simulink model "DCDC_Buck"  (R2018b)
settings: Solver=FixedStepDiscrete  StartTime=0.0  StopTime=Inf  RelTol=1e-3  EnableMultiTasking=on
undefined symbols (not defined in the file): A, ADCIN0, ADCIN1, ADCINA0, ADCINB0, bit, Compare, conversion, DCAEVT1, DCAEVT1FILT, Digital, ended, Event, Filtered, GPTRIP1SEL, GPTRIP2SEL, hex2dec, input, Module, of, Single, start, Trip, TZ1, TZ2, version, Zone
libraries: c2837xDlib x3, c2802xlib x3, tiiqmathlib x2, c280xlib x2, c2000lib x1, demo_controls x1, simulink x1

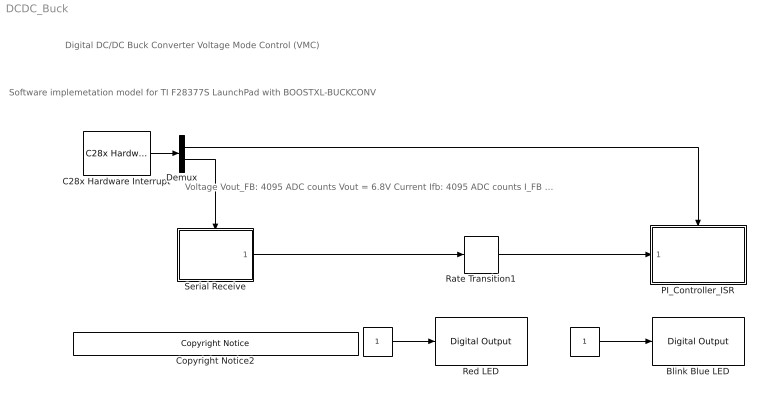
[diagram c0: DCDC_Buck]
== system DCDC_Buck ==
  note: Voltage Vout_FB: 4095 ADC counts Vout = 6.8V Current Ifb: 4095 ADC counts I_FB = 3.3A
  note: Software implemetation model for TI F28377S LaunchPad with BOOSTXL-BUCKCONV
  note: Digital DC/DC Buck Converter Voltage Mode Control (VMC)
  " " : Constant  OutDataTypeStr=uint16  SampleTime=0.5
  "   " : Constant  OutDataTypeStr=uint16  SampleTime=0.5
  Blink Blue LED : c2837xDlib/Digital Output  GPIO_Number=GPIO8~GPIO15  GPIO_Bit0=off  GPIO_BIT0_Toggle=off  GPIO_Bit1=off  GPIO_BIT1_Toggle=off  GPIO_Bit2=off  GPIO_BIT2_Toggle=off  GPIO_Bit3=off  GPIO_BIT3_Toggle=off  GPIO_Bit4=off  GPIO_BIT4_Toggle=on  GPIO_Bit5=on  GPIO_BIT5_Toggle=on  GPIO_Bit6=off  GPIO_BIT6_Toggle=off  GPIO_Bit7=off  GPIO_BIT7_Toggle=off
  C28x Hardware Interrupt : c2000lib/Scheduling/C28x Hardware Interrupt  irqnumbers=[1 9]  pienumbers=[1 1]  irqpriorities=[30 50]  irqpreempts=[0 1]  showinput=off  dspchiptype=C280X
  Copyright Notice2 : demo_controls/Copyright Notice  year=2017  prod=tic2000
  Demux : Demux  Outputs=2
  PI_Controller_ISR : Subsystem
  Rate Transition1 : RateTransition  Integrity=off
  Red LED : c2837xDlib/Digital Output  GPIO_Number=GPIO8~GPIO15  GPIO_Bit0=off  GPIO_BIT0_Toggle=off  GPIO_Bit1=off  GPIO_BIT1_Toggle=off  GPIO_Bit2=off  GPIO_BIT2_Toggle=off  GPIO_Bit3=off  GPIO_BIT3_Toggle=off  GPIO_Bit4=on  GPIO_BIT4_Toggle=off  GPIO_Bit5=off  GPIO_BIT5_Toggle=on  GPIO_Bit6=off  GPIO_BIT6_Toggle=off  GPIO_Bit7=off  GPIO_BIT7_Toggle=off
  Serial Receive : Subsystem  SystemSampleTime=1e-3
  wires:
  Serial Receive/1(Out1) -> Rate Transition1/1
  " "/1 -> Blink Blue LED/1
  Demux/1 -> PI_Controller_ISR/Trigger
  Demux/2 -> Serial Receive/Trigger
  C28x Hardware Interrupt/1 -> Demux/1
  Rate Transition1/1 -> PI_Controller_ISR/1(Voltage/P/I Demand)
  "   "/1 -> Red LED/1

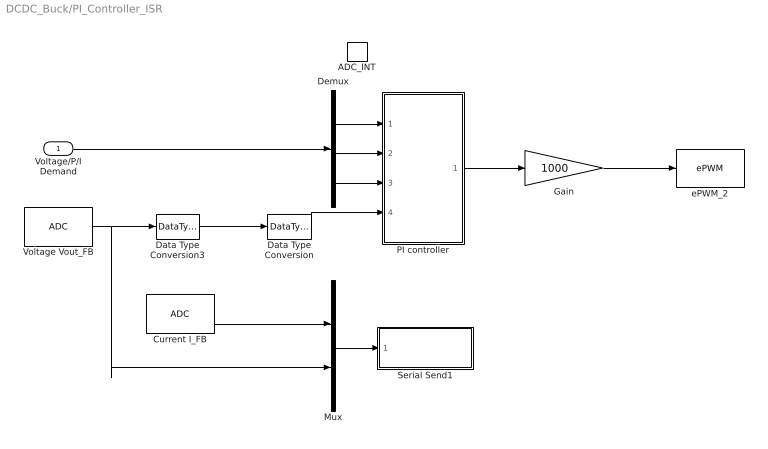
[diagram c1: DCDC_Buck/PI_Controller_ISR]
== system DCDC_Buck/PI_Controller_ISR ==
  Voltage/P/I Demand : Inport
  ADC_INT : TriggerPort  TriggerType=function-call  VariantControl=Variant  PortDimensions=1
  Current I_FB : c2802xlib/ADC  ADCModule=A  samplingMode=Single sample mode  ADCResolution=12-bit (Single-ended input)  useSOC1=SOC1  useSOC2=SOC0_SOC1  SOCAcquisitionWindow=14  SOCTriggerSource=ePWM2_ADCSOCA  SOCInterruptTrigger=No ADCINT  Ts=-1  dType=uint16  postInterrupt=off  interruptSel=ADCINT1  ADCINTContinuous=on  endma=off  chdma=1  blkParamProc=C2000_Type4  conv1=ADCINA0  conv2=ADCINA0 and ADCINB0  conv1_Type4=ADCIN2  conv2_Type4=ADCIN0 and ADCIN1
  Data Type Conversion : DataTypeConversion  OutDataTypeStr=fixdt(1,32,24)  RndMeth=Simplest
  Data Type Conversion3 : DataTypeConversion  OutDataTypeStr=fixdt(0,16,12)  ConvertRealWorld=Stored Integer (SI)  RndMeth=Simplest
  Demux : Demux  Outputs=3
  Gain : Gain  Gain=1000  ParamDataTypeStr=int16  OutDataTypeStr=fixdt(1,32,20)  RndMeth=Simplest
  Mux : Mux  Inputs=2
  PI controller : Subsystem
  Serial Send1 : Subsystem
  Voltage Vout_FB : c2802xlib/ADC  ADCModule=A  samplingMode=Single sample mode  ADCResolution=12-bit (Single-ended input)  useSOC1=SOC0  useSOC2=SOC0_SOC1  SOCAcquisitionWindow=14  SOCTriggerSource=ePWM2_ADCSOCA  SOCInterruptTrigger=No ADCINT  Ts=-1  dType=uint16  postInterrupt=on  interruptSel=ADCINT1  ADCINTContinuous=on  endma=off  chdma=1  blkParamProc=C2000_Type4  conv1=ADCINA0  conv2=ADCINA0 and ADCINB0  conv1_Type4=ADCIN3  conv2_Type4=ADCIN0 and ADCIN1
  ePWM_2 : c2802xlib/ePWM  useModule=ePWM2  ePWMxLINKTBPRD=Not Linked  periodUnits=Clock cycles  timerSource=Specify via dialog  timerPeriod_clk=1000  timerPeriod_sec=0.0001  tbshadow=Counter equals to zero  countingMode=Up  phaseActiveEnable=Disable  phaseDirection=Count down after sync  phaseActive=0  synchronizationEnable=off  dcaevt1Sync=off  dcbevt1Sync=off  synchronizationOption=Disable  clockPrescale=1  HSclockPrescale=1  enswap=off  ePWMxAStatus=on  ePWMxAactionLogic1=Set  ePWMxAactionLogic2=Do nothing  ePWMxAactionLogic3=Clear  ePWMxAactionLogic4=Set  ePWMxAactionLogic5=Do nothing  ePWMxAactionLogic6=Do nothing  ePWMxALoadMode=Load on counter equals to period (CTR=PRD)  ePWMxACSFenable=off  ePWMxACSFvalue=Forcing disable  ePWMxASFreload=Zero  ePWMxBStatus=off  ePWMxBactionLogic1=Set  ePWMxBactionLogic2=Clear  ePWMxBactionLogic3=Do nothing  ePWMxBactionLogic4=Do nothing  ePWMxBactionLogic5=Clear  ePWMxBactionLogic6=Set  ePWMxBLoadMode=Load on counter equals to zero (CTR=Zero)  ePWMxBCSFenable=off  ePWMxBCSFvalue=Forcing disable  ePWMxBSFreload=Zero  ePWNxBOutWay=off  ePWMxLINKCMPA=Not Linked  CMPAUnits=Clock cycles  CMPASource=Input port  CMPAValue_per=50  CMPAValue_clk=0  enCMPAshadow=Counter equals to zero  ePWMxLINKCMPB=Not Linked  CMPBUnits=Clock cycles  CMPBSource=Specify via dialog  CMPBValue_per=50  CMPBValue_clk=1000-((15+54)*2)  enCMPBshadow=Counter equals to zero  ePWMxLINKCMPC=Not Linked  CMPCUnits=Clock cycles  CMPCSource=Specify via dialog  CMPCValue_per=50  CMPCValue_clk=32000  enCMPCshadow=Counter equals to zero  ePWMxLINKCMPD=Not Linked  CMPDUnits=Clock cycles  CMPDSource=Specify via dialog  CMPDValue_per=50  CMPDValue_clk=32000  enCMPDshadow=Counter equals to zero  enableDBePWMxA=on  enableDBePWMxB=on  enhalfcycle=off  DBpolarity=Active high complementary (AHC)  DBedgeDelay=Positive  DBSource_ePWMxA=ePWMxA  DBSource_ePWMxB=ePWMxA  DBperiodSource=Specify via dialog  REDperiod=20  FEDperiod=20  adcstartModuleA=on  adcrequestEventA=First event  adcstartEventA=Digital Compare Module A Event 1 start of conversion (DCAEVT1.soc)  adcstartEventA_type2=Counter is incrementing and equals to the compare B register (CTRU=CMPB)  adcstartModuleB=off  adcrequestEventB=First event  adcstartEventB=Counter equals to zero (CTR=Zero)  adcstartEventB_type2=Counter equals to zero (CTR=Zero)  intEn=off  intPrd=First event  intSel=Counter equals to zero (CTR=Zero)  intSel_type2=Counter equals to zero (CTR=Zero)  hrpe=off  enHRPWM=off  HRPWM_LoadMode=Counter equals to period (CTR=PRD)  HRPWM_CTLMode=Duty or Period control mode  HRPWM_EDGMode=Both edge  hrpeb=off  enHRPWMB=off  HRPWM_LoadModeB=Counter equals to zero (CTR=ZERO)  HRPWM_CTLModeB=Duty or Period control mode  HRPWM_EDGModeB=Both edge  enSFO=on  enautoconv=on  chopperEnable=off  chopperFrequency=1  chopperFirstwidth=1  chopperDuty=12.5%  tripZonesource=Specify via dialog  tzselOSHT1=off  tzselOSHT2=off  tzselOSHT3=off  tzselOSHDCAEV1=off  tzselOSHDCBEV1=off  tzselCBC1=off  tzselCBC2=off  tzselCBC3=off  tzselCBCDCAEV2=off  tzselCBCDCBEV2=off  tzselOSHT4=off  tzselOSHT5=off  tzselOSHT6=off  tzselCBC4=off  tzselCBC5=off  tzselCBC6=off  enTzOstIntr=off  enTzCbcIntr=off  enTzDCAEVT1Intr=off  enTzDCAEVT2Intr=off  enTzDCBEVT1Intr=off  enTzDCBEVT2Intr=off  ePWMxAforced=No action  ePWMxBforced=No action  DCAEVT1forced=No action  DCBEVT1forced=No action  DCAEVT2forced=No action  DCBEVT2forced=No action  dcah=Trip Zone 1 input (TZ1)  dcal=Trip Zone 2 input (TZ2)  dcbh=Trip Zone 1 input (TZ1)  dcbl=Trip Zone 2 input (TZ2)  dcah_type2=GPTRIP1SEL/(TZ1)  dcal_type2=GPTRIP2SEL/(TZ2)  dcbh_type2=GPTRIP1SEL/(TZ1)  dcbl_type2=GPTRIP2SEL/(TZ2)  gendcaevt1=Event disabled  gendcaevt2=Event disabled  gendcbevt1=Event disabled  gendcbevt2=Event disabled  dcaevt1src=DCAEVT1 with sync  dcaevt2src=DCAEVT2 with sync  dcbevt1src=DCBEVT1 with sync  dcbevt2src=DCBEVT2 with sync  pulsesel=Counter equals to zero (CTR=Zero)  blankinv=off  blankoffset=0  blankwidth=0  evsrcsel=Filtered version of DCAEVT1 (DCAEVT1FILT)  encape=off  PwmType=C2000_Type4
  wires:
  Data Type Conversion3/1 -> Data Type Conversion/1
  Gain/1 -> ePWM_2/1
  PI controller/1(Duty1) -> Gain/1
  Data Type Conversion/1 -> PI controller/4(Vout1)
  Mux/1 -> Serial Send1/1(In1)
  Demux/1 -> PI controller/1(Vout1Ref)
  Demux/2 -> PI controller/2(P gain)
  Demux/3 -> PI controller/3(I gain)
  Voltage/P/I Demand/1 -> Demux/1
  Current I_FB/1 -> Mux/1
  Voltage Vout_FB/1 -> Mux/2, Data Type Conversion3/1

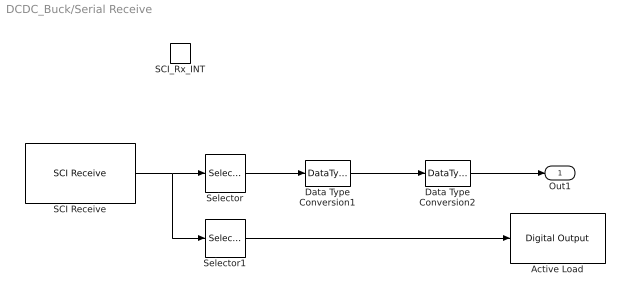
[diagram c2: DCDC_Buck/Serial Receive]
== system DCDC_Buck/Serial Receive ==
  SCI_Rx_INT : TriggerPort  TriggerType=function-call  VariantControl=Variant
  Active Load : c2837xDlib/Digital Output  GPIO_Number=GPIO16~GPIO23  GPIO_Bit0=off  GPIO_BIT0_Toggle=off  GPIO_Bit1=off  GPIO_BIT1_Toggle=off  GPIO_Bit2=on  GPIO_BIT2_Toggle=off  GPIO_Bit3=off  GPIO_BIT3_Toggle=off  GPIO_Bit4=off  GPIO_BIT4_Toggle=on  GPIO_Bit5=off  GPIO_BIT5_Toggle=off  GPIO_Bit6=off  GPIO_BIT6_Toggle=off  GPIO_Bit7=off  GPIO_BIT7_Toggle=off
  Data Type Conversion1 : DataTypeConversion  OutDataTypeStr=fixdt(0,16,14)  ConvertRealWorld=Stored Integer (SI)  RndMeth=Simplest
  Data Type Conversion2 : DataTypeConversion  OutDataTypeStr=fixdt(1,32,24)  RndMeth=Simplest
  SCI Receive : c280xlib/SCI Receive  sciModule=A  dataHead='S'  dataTail='E'  dataType=uint16  dataDim=4  initValue=0  errOption=Output the last received value  errValue=0  sampleTime=-1  outputStatus=off  postInterrupt=on  numFifo=10
  Selector : Selector  InputPortWidth=4  IndexOptions=Index vector (dialog)  Indices=[1 2 3]  OutputSizes=1
  Selector1 : Selector  InputPortWidth=4  IndexOptions=Index vector (dialog)  Indices=4  OutputSizes=1
  Out1 : Outport  InitialOutput=[0 0.002 0.003]
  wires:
  SCI Receive/1 -> Selector1/1, Selector/1
  Selector/1 -> Data Type Conversion1/1
  Selector1/1 -> Active Load/1
  Data Type Conversion1/1 -> Data Type Conversion2/1
  Data Type Conversion2/1 -> Out1/1

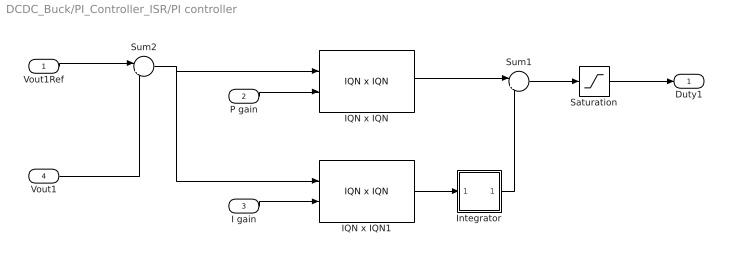
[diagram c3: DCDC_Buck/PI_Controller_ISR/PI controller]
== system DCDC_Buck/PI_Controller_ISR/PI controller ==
  Vout1Ref : Inport
  P gain : Inport  Port=2
  I gain : Inport  Port=3
  Vout1 : Inport  Port=4
  IQN x IQN : tiiqmathlib/IQN x IQN  multiplyOption=Multiply
  IQN x IQN1 : tiiqmathlib/IQN x IQN  multiplyOption=Multiply
  Integrator : Subsystem
  Saturation : Saturate  UpperLimit=0.6  LowerLimit=0  RndMeth=Simplest
  Sum1 : Sum  Inputs=|++  RndMeth=Simplest
  Sum2 : Sum  Inputs=|+-  RndMeth=Simplest
  Duty1 : Outport
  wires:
  P gain/1 -> IQN x IQN/2
  Vout1Ref/1 -> Sum2/1
  Integrator/1(y) -> Sum1/2
  Vout1/1 -> Sum2/2
  Sum2/1 -> IQN x IQN/1, IQN x IQN1/1
  I gain/1 -> IQN x IQN1/2
  Sum1/1 -> Saturation/1
  Saturation/1 -> Duty1/1
  IQN x IQN/1 -> Sum1/1
  IQN x IQN1/1 -> Integrator/1(u)

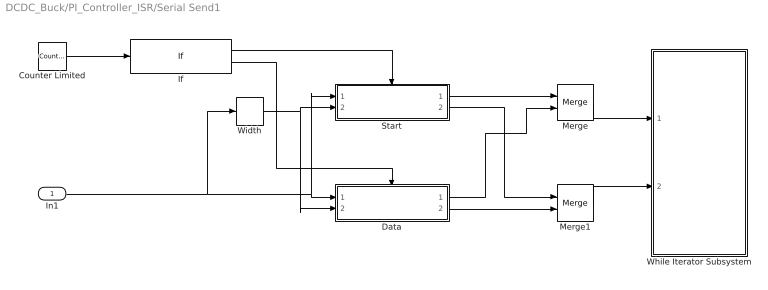
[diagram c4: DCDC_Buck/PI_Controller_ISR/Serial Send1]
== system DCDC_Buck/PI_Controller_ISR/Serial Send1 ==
  In1 : Inport
  Counter Limited : simulink/Sources/Counter Limited  uplimit=11999  tsamp=-1
  Data : Subsystem  TreatAsAtomicUnit=on
  If : If  IfExpression=u1 == 0
  Merge : Merge
  Merge1 : Merge
  Start : Subsystem  TreatAsAtomicUnit=on
  While Iterator Subsystem : Subsystem  TreatAsAtomicUnit=on
  Width : Width  OutDataTypeMode=All ports same datatype  DataType=uint16
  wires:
  If/1 -> Start/Action
  If/2 -> Data/Action
  Counter Limited/1 -> If/1
  Start/1(Data_out) -> Merge/1
  Data/1(Data_out) -> Merge/2
  Merge/1 -> While Iterator Subsystem/1(Data)
  Merge1/1 -> While Iterator Subsystem/2(Iteration)
  Start/2(Iteration) -> Merge1/1
  Data/2(Iteration) -> Merge1/2
  Width/1 -> Data/2(Data_width), Start/2(Data_width)
  In1/1 -> Width/1, Start/1(Data), Data/1(Data)

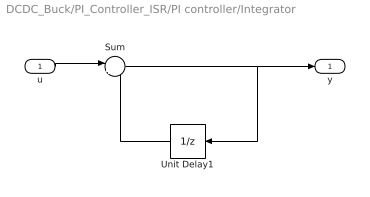
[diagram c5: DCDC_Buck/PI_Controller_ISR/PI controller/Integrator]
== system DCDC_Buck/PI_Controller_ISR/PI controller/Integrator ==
  u : Inport
  Sum : Sum  Inputs=|++  RndMeth=Simplest
  Unit Delay1 : UnitDelay  SampleTime=-1
  y : Outport
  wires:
  Sum/1 -> Unit Delay1/1, y/1
  Unit Delay1/1 -> Sum/2
  u/1 -> Sum/1

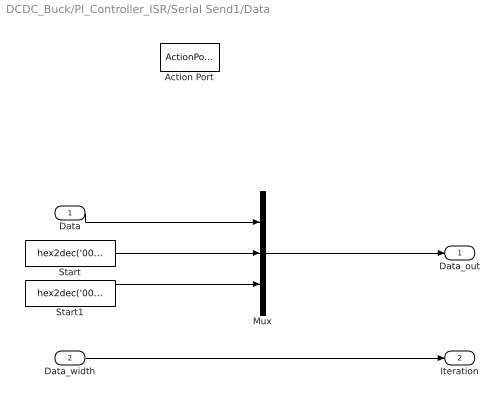
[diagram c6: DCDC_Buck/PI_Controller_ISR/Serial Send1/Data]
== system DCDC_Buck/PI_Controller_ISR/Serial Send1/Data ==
  Data : Inport
  Data_width : Inport  Port=2
  Action Port : ActionPort  ActionType=else
  Mux : Mux  Inputs=3
  Start : Constant  Value=hex2dec('0000')  OutDataTypeStr=uint16
  Start1 : Constant  Value=hex2dec('0000')  OutDataTypeStr=uint16
  Data_out : Outport
  Iteration : Outport  Port=2
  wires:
  Start/1 -> Mux/2
  Mux/1 -> Data_out/1
  Data/1 -> Mux/1
  Data_width/1 -> Iteration/1
  Start1/1 -> Mux/3

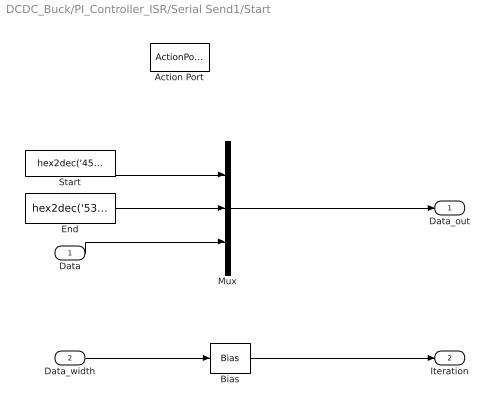
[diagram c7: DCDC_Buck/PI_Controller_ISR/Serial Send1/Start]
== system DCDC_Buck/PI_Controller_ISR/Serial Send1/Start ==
  Data : Inport
  Data_width : Inport  Port=2
  Action Port : ActionPort  ActionType=then
  Bias : Bias  Bias=2
  End : Constant  Value=hex2dec('5353')  OutDataTypeStr=uint16
  Mux : Mux  Inputs=3
  Start : Constant  Value=hex2dec('4545')  OutDataTypeStr=uint16
  Data_out : Outport
  Iteration : Outport  Port=2
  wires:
  End/1 -> Mux/2
  Mux/1 -> Data_out/1
  Data_width/1 -> Bias/1
  Bias/1 -> Iteration/1
  Data/1 -> Mux/3
  Start/1 -> Mux/1

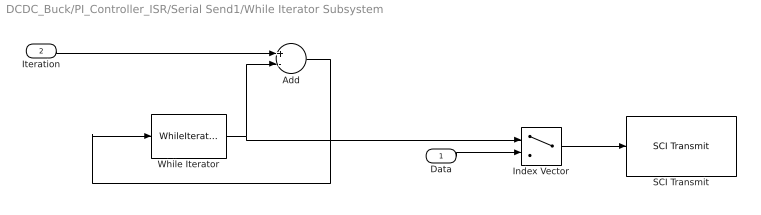
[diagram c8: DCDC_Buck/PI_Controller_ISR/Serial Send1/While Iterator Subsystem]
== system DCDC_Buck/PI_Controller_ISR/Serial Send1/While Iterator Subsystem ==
  Data : Inport
  Iteration : Inport  Port=2
  Add : Sum  Inputs=+-
  Index Vector : MultiPortSwitch  Inputs=1
  SCI Transmit : c280xlib/SCI Transmit  sciModule=A  dataHead=''  dataTail=''  postInterrupt=off  numFifo=1
  While Iterator : WhileIterator  MaxIters=-1  WhileBlockType=do-while  ShowIterationPort=on  OutputDataType=int16
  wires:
  Iteration/1 -> Add/1
  Add/1 -> While Iterator/1
  Index Vector/1 -> SCI Transmit/1
  Data/1 -> Index Vector/2
  While Iterator/1 -> Index Vector/1, Add/2
